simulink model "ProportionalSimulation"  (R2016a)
settings: Solver=VariableStepAuto  StartTime=0.0  StopTime=10.0  RelTol=1e-3
libraries: vexarmcortexlib x5, simulink x1

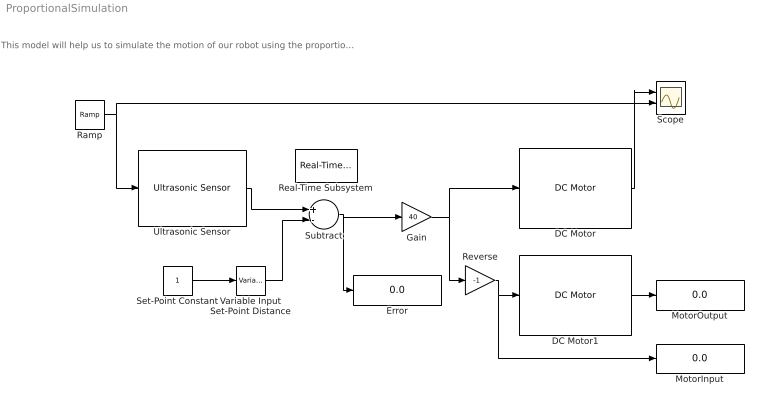
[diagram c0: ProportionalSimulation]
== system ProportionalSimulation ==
  note: This model will help us to simulate the motion of our robot using the proportional controller.
  DC Motor : vexarmcortexlib/DC Motor  motor=3  scaleFactor=1/13.5  SimulationOut=on
  DC Motor1 : vexarmcortexlib/DC Motor  motor=7  scaleFactor=1/13.5  SimulationOut=on
  Error : Display
  Gain : Gain  Gain=40
  MotorInput : Display
  MotorOutput : Display
  Ramp : simulink/Sources/Ramp  slope=1  start=0  X0=0
  Real-Time Subsystem : vexarmcortexlib/Utilities/Real-Time Subsystem  x=1
  Reverse : Gain  Gain=-1
  Scope : Scope  NumInputPorts=2
  Set-Point Constant : Constant
  Subtract : Sum  Inputs=+-
  Ultrasonic Sensor : vexarmcortexlib/Ultrasonic Sensor  inputPin=3  outputPin=2  inputPortSim=on  SampleTime=0.2
  Variable Input Set-Point Distance : vexarmcortexlib/Utilities/Variable Input  low=0  gain=0.2  high=2
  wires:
  Ultrasonic Sensor/1 -> Subtract/1
  Subtract/1 -> Error/1, Gain/1
  Gain/1 -> DC Motor/1, Reverse/1
  Reverse/1 -> MotorInput/1, DC Motor1/1
  Variable Input Set-Point Distance/1 -> Subtract/2
  Set-Point Constant/1 -> Variable Input Set-Point Distance/1
  DC Motor1/1 -> MotorOutput/1
  Ramp/1 -> Ultrasonic Sensor/1, Scope/2
  DC Motor/1 -> Scope/1
